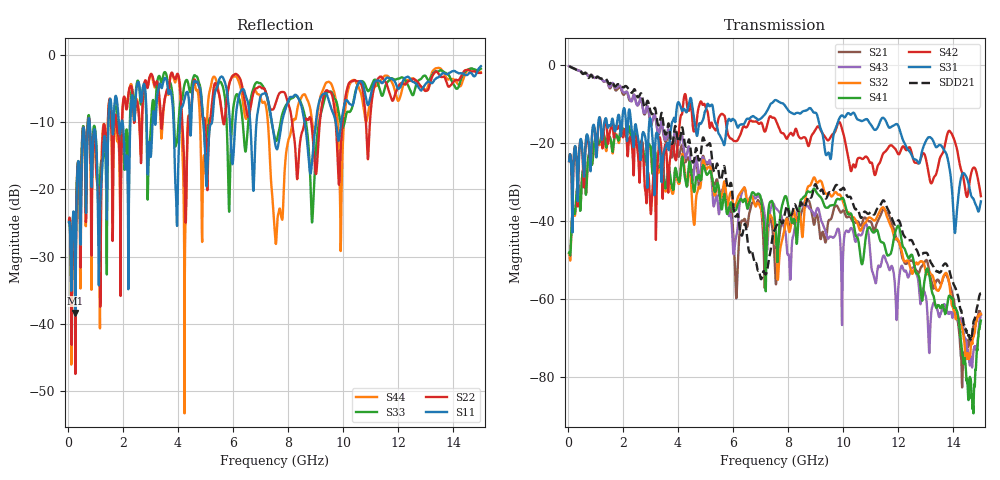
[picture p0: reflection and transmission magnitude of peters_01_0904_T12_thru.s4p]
# MHZ S RI R 50.00
! FREQ  S11  S12  S13  S14
!  S21  S22  S23  S24
!  S31  S32  S33  S34
!  S41  S42  S43  S44
!  REAL  IMAG  REAL  IMAG  REAL  IMAG  REAL  IMAG
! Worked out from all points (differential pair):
!   1496 points, 50 MHz to 15 GHz, reference 50 ohm
!   strongest paths, dB at 50 MHz, 3.79 GHz, 7.53 GHz, 11.27 GHz, 15 GHz:
!     S31: -24.8, -14.8, -9.1, -15.9, -35.1
!     S42: -24.8, -20.5, -13.9, -25.8, -33.8
!     S41: -48.2, -31.5, -40.7, -43.1, -65.6
!     S32: -48.5, -32.9, -44.1, -38.5, -64.0
!     S43: -0.4, -21.7, -36.6, -51.6, -64.1
!     S21: -0.4, -23.8, -52.9, -39.9, -64.2
!   taken as a pair (ports 3,1 in; 4,2 out), SDD21 dB: -0.4, -20.4, -42.1, -36.7, -58.6
!   lowest |S11| = -38.4 dB at 280 MHz (marker M1), VSWR 1.02, Z = 51.2 + j0.315 ohm
!   |S11| at or under -10 dB: start of sweep to 741.2 MHz; 794.5 MHz to 1.474 GHz (679.4 MHz wide, 59.9 % of centre); 8.6 GHz to 9.009 GHz (408.4 MHz wide, 4.64 % of centre)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
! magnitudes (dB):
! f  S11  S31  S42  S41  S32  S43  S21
! 50 MHz  -24.9  -24.8  -24.8  -48.2  -48.5  -0.4  -0.4
! 280 MHz  -38.4  -21.1  -21.2  -37.2  -37.6  -1.2  -1.2
! 5.13 GHz  -11.9  -10.6  -15.0  -27.7  -26.3  -24.7  -24.9
! 6.12 GHz  -8.4  -15.3  -19.6  -37.1  -35.5  -44.0  -59.9
! 7.55 GHz  -13.5  -9.1  -14.2  -42.5  -45.9  -36.8  -55.8
! 11.49 GHz  -3.8  -13.8  -22.5  -46.0  -36.9  -49.0  -37.1
! 15 GHz  -1.6  -35.1  -33.8  -65.6  -64.0  -64.1  -64.2
